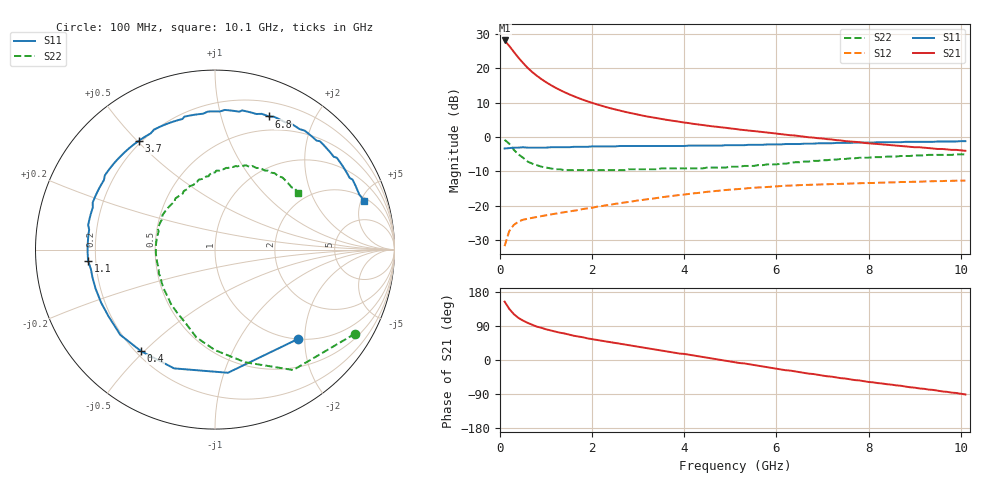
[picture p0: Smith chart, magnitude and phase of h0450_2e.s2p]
!HBFP-0450
!S and NOISE PARAMETERS at Vce=2V  Ic=15mA.  LAST UPDATED  09-04-98
# GHZ S MA R  50
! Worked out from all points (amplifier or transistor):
!   101 points, 100 MHz to 10.1 GHz, reference 50 ohm
!   highest |S21| = 28.0 dB at 100 MHz (marker M1)
!   |S21| within 3 dB of that: start of sweep to 282.2 MHz
!   unconditionally stable (mu >= 1): 2.45 GHz to 2.59 GHz; 2.605 GHz to end of sweep
!   at 1.7 GHz: K = 0.85, MSG = 16.3 dB, |S12| = -21.2 dB
!   at 5.1 GHz: K = 1.12, MAG = 6.7 dB, |S12| = -15.2 dB
!   at 10.1 GHz: K = 1.05, MAG = 2.9 dB, |S12| = -12.7 dB
!   lowest NFmin = 1.23 dB at 1.8 GHz
!   S11 on the Smith chart (normalised r, x): 100 MHz: 1.01, -1.86; 400 MHz: 0.22, -0.49; 1.1 GHz: 0.17, -0.04; 3.7 GHz: 0.19, +0.51; 6.8 GHz: 0.35, +1.43; 10.1 GHz: 2.38, +5.27
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0.1  0.68 -47.0  25.19 154.0  0.026 69.0  0.91 -31.0
0.2  0.69 -84.0  21.02 135.0  0.043 53.0  0.8 -57.0
0.3  0.7 -109.0  17.21 121.0  0.053 43.0  0.65 -75.0
0.4  0.7 -126.0  14.17 111.0  0.059 37.0  0.56 -90.0
0.5  0.71 -138.0  11.88 104.0  0.063 33.0  0.5 -102.0
0.6  0.7 -148.0  10.07 98.0  0.065 31.0  0.44 -112.0
0.7  0.7 -155.0  8.76 93.0  0.067 29.0  0.41 -121.0
0.8  0.7 -162.0  7.73 88.0  0.069 28.0  0.39 -129.0
0.9  0.7 -167.0  6.91 85.0  0.071 27.0  0.37 -136.0
1  0.7 -171.0  6.24 81.0  0.073 27.0  0.36 -142.0
1.1  0.71 -175.0  5.68 78.0  0.075 27.0  0.35 -148.0
1.4  0.71 174.0  4.47 70.0  0.081 26.0  0.33 -162.0
1.6  0.72 169.0  3.91 64.0  0.085 26.0  0.33 -169.0
1.8  0.72 164.0  3.47 60.0  0.09 25.0  0.33 -176.0
2.1  0.73 156.0  2.98 53.0  0.097 25.0  0.33 175.0
2.5  0.73 148.0  2.51 45.0  0.107 23.0  0.33 166.0
3.5  0.74 128.0  1.83 25.0  0.133 16.0  0.35 147.0
3.7  0.74 125.0  1.74 21.0  0.138 14.0  0.35 143.0
5.1  0.76 99.0  1.31 -6.0  0.174 -2.0  0.37 116.0
6.8  0.8 68.0  0.98 -37.0  0.203 -25.0  0.45 85.0
8.5  0.84 41.0  0.76 -65.0  0.219 -46.0  0.52 60.0
10.1  0.87 18.0  0.63 -91.0  0.233 -69.0  0.56 34.0
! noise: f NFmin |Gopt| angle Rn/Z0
1.8  1.23  0.45  -173  0.06
2  1.27  0.47  -169  0.06
2.5  1.41  0.52  -156  0.07
3.5  1.66  0.61  -136  0.16
4  1.81  0.64  -124  0.26
5  2.08  0.69  -103  0.55
5.5  2.22  0.72  -93  0.79
7  2.62  0.76  -65  1.8
8  2.89  0.81  -48  2.73
10  3.42  0.83  -18  4.67
